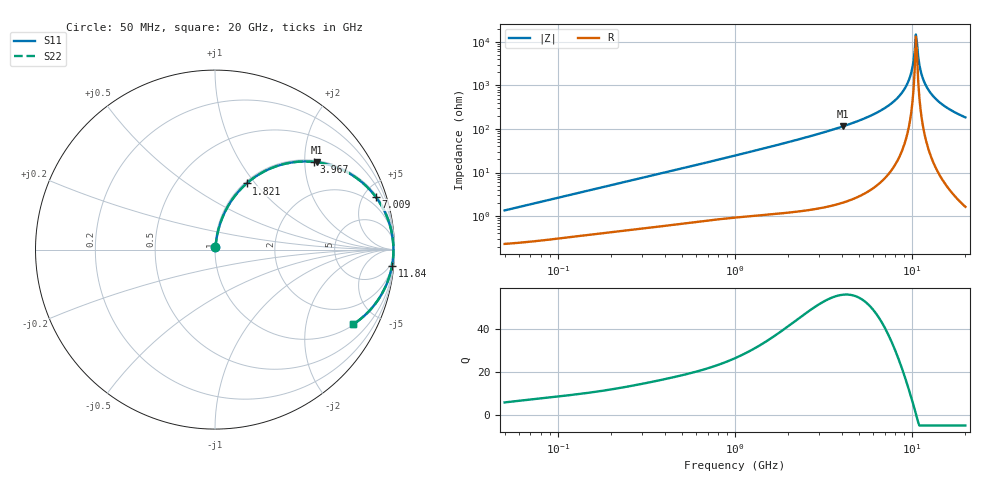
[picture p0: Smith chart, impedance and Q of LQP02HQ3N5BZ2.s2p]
!Murata Part Number: LQP02HQ3N5BZ2
!These Parameters are Measured in Series Mode Connection
!  o--[Z]--o
!Port1  Port2
!  o-------o
!Freq. Start=50[MHz] Stop=20[GHz], 401[Steps]
# Hz S RI R 50
!Freq.(Hz) S11(Real) S11(Imag) S21(Real) S21(Imag) S12(Real) S12(Imag) S22(Real) S22(Imag)
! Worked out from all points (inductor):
!   401 points, 50 MHz to 20 GHz, reference 50 ohm
!   read as one part in series: L = 4.22 nH near 51.52 MHz
!   highest Q = 56.2 at 4.088 GHz (marker M1), where L = 4.5 nH
!   self-resonance near 10.5 GHz
!   S11 on the Smith chart (normalised r, x): 50 MHz: 1.00, +0.03; 1.821 GHz: 1.02, +0.90; 3.967 GHz: 1.04, +2.22; 7.009 GHz: 1.15, +6.02; 11.84 GHz: 2, -22; 20 GHz: 1.03, -3.69
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5e7  0.00248 0.0133  0.9975 -0.0133  0.9975 -0.0133  0.00248 0.0133
1.364002e8  0.00477 0.0349  0.9952 -0.0349  0.9952 -0.0349  0.00477 0.0349
3.721004e8  0.0141 0.091  0.9859 -0.091  0.9859 -0.091  0.0141 0.091
1e9  0.0644 0.2273  0.9356 -0.2273  0.9356 -0.2273  0.0644 0.2273
1.820564e9  0.1761 0.3683  0.8239 -0.3683  0.8239 -0.3683  0.1761 0.3683
2.728004e9  0.3338 0.4616  0.6662 -0.4616  0.6662 -0.4616  0.3338 0.4616
3.967106e9  0.5508 0.4886  0.4492 -0.4886  0.4492 -0.4886  0.5508 0.4886
4.087748e9  0.5702 0.4862  0.4298 -0.4862  0.4298 -0.4862  0.5702 0.4862
5.515528e9  0.7642 0.4151  0.2358 -0.4151  0.2358 -0.4151  0.7642 0.4151
7.009217e9  0.8949 0.2946  0.1051 -0.2946  0.1051 -0.2946  0.8949 0.2946
7.442007e9  0.9207 0.2568  0.0793 -0.2568  0.0793 -0.2568  0.9207 0.2568
8.516016e9  0.9655 0.1632  0.0345 -0.1632  0.0345 -0.1632  0.9655 0.1632
9.316812e9  0.9842 0.0959  0.0158 -0.0959  0.0158 -0.0959  0.9842 0.0959
9.892087e9  0.9913 0.0498  0.00871 -0.0498  0.00871 -0.0498  0.9913 0.0498
1.034674e10  0.9937 0.0148  0.00627 -0.0148  0.00627 -0.0148  0.9937 0.0148
1.050288e10  0.994 0.00306  0.006 -0.00306  0.006 -0.00306  0.994 0.00306
1.082228e10  0.9937 -0.0203  0.00631 0.0203  0.00631 0.0203  0.9937 -0.0203
1.131968e10  0.9911 -0.0554  0.00885 0.0554  0.00885 0.0554  0.9911 -0.0554
1.183995e10  0.9861 -0.0901  0.0139 0.0901  0.0139 0.0901  0.9861 -0.0901
1.276073e10  0.9724 -0.1468  0.0276 0.1468  0.0276 0.1468  0.9724 -0.1468
1.438523e10  0.937 -0.2327  0.063 0.2327  0.063 0.2327  0.937 -0.2327
2e10  0.7711 -0.4157  0.2289 0.4157  0.2289 0.4157  0.7711 -0.4157
